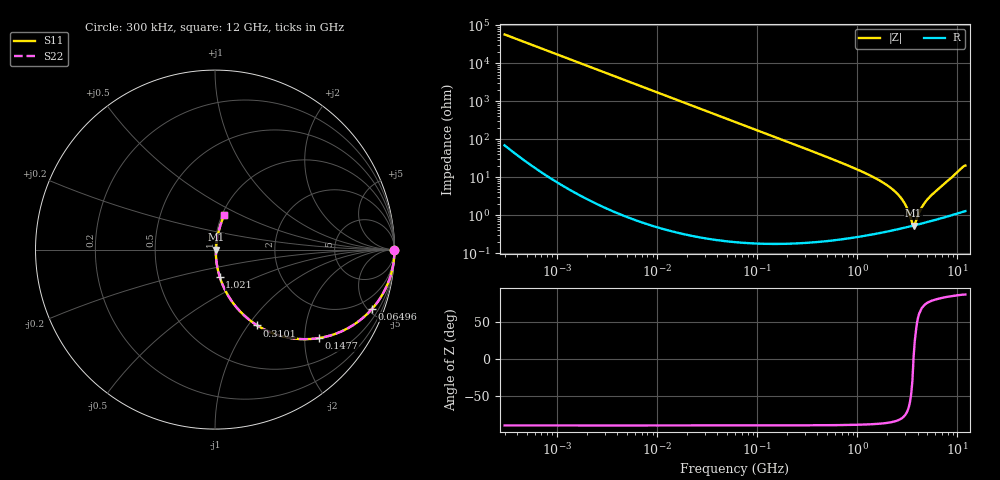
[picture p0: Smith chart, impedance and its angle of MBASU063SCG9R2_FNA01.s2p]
! MBASU063SCG9R2_FNA01  S-PARAMETER MODEL  ( General Type )
! Model Generated by TAIYO YUDEN Corporation (http://www.ty-top.com)
! Version 1.0
! TAIYO YUDEN Control No. 130801
! Copyright(c) 2013 TAIYO YUDEN CO.,LTD. All Rights Reserved.
! Product Description (link to TY-COMPAS)
! https://ds.yuden.co.jp/TYCOMPAS/or/detail?pn=MBASU063SCG9R2DFNA01&u=M
! Products Name : Multilayer Ceramic Capacitors
! Characteristics :
!  Capacitance : 9.2 pF , Rated Voltage : 50V , TCC : CG / C0G
!  Case Size : 0.6 x 0.3 / 0.024 x 0.012 [mm/inch] , Thickness : 0.3 / 0.012 [mm/inch]
!  (Conditions: Temperature = 25 degC , DC Bias Current/Voltage = 0A / 0V)
! External Node Assignments :
!  1  o---| |---o  2
! GND o---------o GND
! Frequency Range : 0.3MHz  -  12000MHz  [ 401 STEP ]
# MHz S RI R 50
! Freq[MHz].  S11 Real  S11 Imag  S21 Real  S21 Imag  S12 Real  S12 Imag  S22 Real  S22 Imag
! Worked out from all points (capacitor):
!   401 points, 300 kHz to 12 GHz, reference 50 ohm
!   read as one part in series: C = 9.21 pF near 316.3 kHz
!   lowest |Z| = 534 mohm at 3.643 GHz (marker M1)
!   series resonance near 3.639 GHz, so ESL is about 210 pH
!   S11 on the Smith chart (normalised r, x): 300 kHz: open; 64.96 MHz: 1.00, -5.32; 147.7 MHz: 1.00, -2.34; 310.1 MHz: 1.00, -1.11; 1.021 GHz: 1.01, -0.31; 12 GHz: 1.03, +0.41
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0.3  1 -0.00174  5.1e-06 0.00174  5.1e-06 0.00174  1 -0.00174
1.769972  0.9999 -0.0102  0.000108 0.0102  0.000108 0.0102  0.9999 -0.0102
10.44266  0.9963 -0.0602  0.00366 0.0602  0.00366 0.0602  0.9963 -0.0602
26.39317  0.9771 -0.1492  0.0229 0.1492  0.0229 0.1492  0.9771 -0.1492
60  0.8922 -0.3098  0.1078 0.3098  0.1078 0.3098  0.8922 -0.3098
64.96309  0.8759 -0.3293  0.1241 0.3293  0.1241 0.3293  0.8759 -0.3293
147.6816  0.577 -0.4933  0.423 0.4933  0.423 0.4933  0.577 -0.4933
310.0777  0.2351 -0.4224  0.7649 0.4224  0.7649 0.4224  0.2351 -0.4224
353.9943  0.1905 -0.3907  0.8095 0.3907  0.8095 0.3907  0.1905 -0.3907
570.2811  0.0821 -0.2708  0.9179 0.2708  0.9179 0.2708  0.0821 -0.2708
1021.415  0.0263 -0.1515  0.9737 0.1515  0.9737 0.1515  0.0263 -0.1515
2088.533  0.00688 -0.0552  0.9931 0.0552  0.9931 0.0552  0.00688 -0.0552
2514.07  0.00553 -0.036  0.9945 0.036  0.9945 0.036  0.00553 -0.036
2870.14  0.00511 -0.023  0.9949 0.023  0.9949 0.023  0.00511 -0.023
3107.553  0.00504 -0.0154  0.995 0.0154  0.995 0.0154  0.00504 -0.0154
3454.93  0.00517 -0.00543  0.9948 0.00543  0.9948 0.00543  0.00517 -0.00543
3642.919  0.00531 0.000119  0.9947 -0.000119  0.9947 -0.000119  0.00531 0.000119
3841.137  0.00552 0.00408  0.9945 -0.00408  0.9945 -0.00408  0.00552 0.00408
4502.883  0.00638 0.0164  0.9936 -0.0164  0.9936 -0.0164  0.00638 0.0164
5140.631  0.00742 0.0269  0.9926 -0.0269  0.9926 -0.0269  0.00742 0.0269
8281.503  0.0168 0.0846  0.9832 -0.0846  0.9832 -0.0846  0.0168 0.0846
12000  0.0508 0.1903  0.9492 -0.1903  0.9492 -0.1903  0.0508 0.1903
